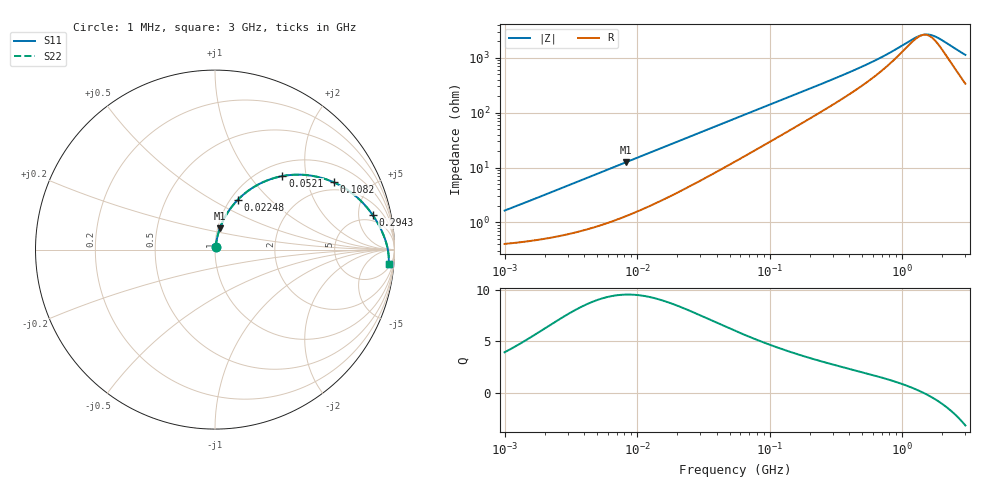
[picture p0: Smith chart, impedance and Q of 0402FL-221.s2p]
# MHz S MA R 50
!Freq  MagS11  AngS11  MagS21  AngS21  MagS12  AngS12  MagS22  AngS22
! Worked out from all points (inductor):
!   801 points, 1 MHz to 3 GHz, reference 50 ohm
!   read as one part in series: L = 252 nH near 1.041 MHz
!   highest Q = 9.54 at 8.18 MHz (marker M1), where L = 240 nH
!   self-resonance near 1.437 GHz
!   S11 on the Smith chart (normalised r, x): 1 MHz: 1.01, +0.03; 22.48 MHz: 1.08, +0.66; 52.1 MHz: 1.24, +1.47; 108.2 MHz: 1.65, +2.94; 294.3 MHz: 3.71, +7.49; 3 GHz: 8, -22
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1  0.01641 74.8  0.9958 -0.9  0.9958 -0.9  0.01641 74.8
3.823119  0.05885 79.8  0.9913 -3.3  0.9913 -3.3  0.05885 79.8
8.179831  0.1216 77.1  0.98 -6.9  0.98 -6.9  0.1216 77.1
14.47069  0.2063 71.9  0.9562 -11.8  0.9562 -11.8  0.2063 71.9
22.47661  0.3032 65.5  0.917 -17.5  0.917 -17.5  0.3032 65.5
33.87922  0.419 57.6  0.8522 -24.5  0.8522 -24.5  0.419 57.6
52.09891  0.5561 47.5  0.7465 -33.3  0.7465 -33.3  0.5561 47.5
54.77226  0.5721 46.2  0.7317 -34.4  0.7317 -34.4  0.5721 46.2
76.20648  0.672 37.9  0.6253 -41.3  0.6253 -41.3  0.672 37.9
108.1723  0.7605 29.5  0.5051 -47.9  0.5051 -47.9  0.7605 29.5
150.5037  0.8233 22.6  0.3978 -52.9  0.3978 -52.9  0.8233 22.6
209.4008  0.8682 16.9  0.3046 -56.2  0.3046 -56.2  0.8682 16.9
294.2768  0.9002 12.3  0.2259 -57.8  0.2259 -57.8  0.9002 12.3
515.4121  0.9333 6.7  0.1305 -56.0  0.1305 -56.0  0.9333 6.7
792.5923  0.949 3.5  0.07889 -48.0  0.07889 -48.0  0.949 3.5
1268.618  0.9607 0.7  0.04113 -17.0  0.04113 -17.0  0.9607 0.7
1402.151  0.9627 0.1  0.03742 -3.6  0.03742 -3.6  0.9627 0.1
1534.307  0.9642 -0.4  0.03636 10.1  0.03636 10.1  0.9642 -0.4
1678.92  0.9657 -0.9  0.03769 23.9  0.03769 23.9  0.9657 -0.9
1855.641  0.9671 -1.5  0.04182 37.3  0.04182 37.3  0.9671 -1.5
2797.026  0.9707 -4.2  0.07786 65.8  0.07786 65.8  0.9707 -4.2
3000  0.9709 -4.7  0.08615 67.9  0.08615 67.9  0.9709 -4.7
